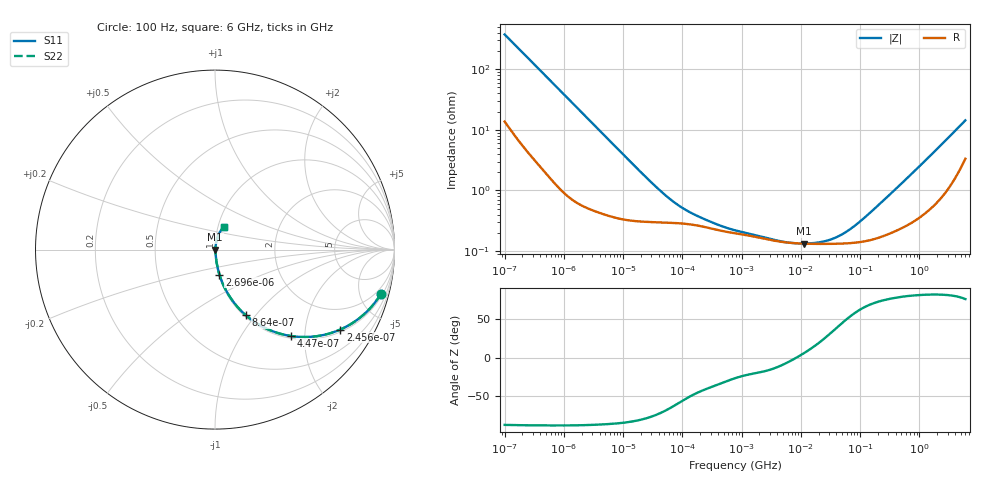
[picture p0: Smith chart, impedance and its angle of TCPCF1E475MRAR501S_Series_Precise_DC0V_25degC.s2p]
! TCPCF1E475MRAR501S Polymer Tantalum Capacitor Sparameter Model
! Model Generated by Samsung Electro-Mechanics
! Samsung Sparameter Version 5.0
! Date : Oct-10-2024
! Products : Polymer Tantalum Capacitor
! Characteristics :
!  Nominal Capacitance = 4.7uF
!  Capacitance Tolerance = +/-20%
!  ESR = 500 mohm max at 100kHz
!  Rated Voltage = 25Vdc
!  Size = 0805(unit:inch), 2012(unit:mm)
!  Length = 2.00+/-0.20mm
!  Width = 1.25+/-0.20mm
!  Thickness = 0.90+/-0.10mm
!  Lineup = Conductive Polymer Type
!  Feature = PCF
!  Measurement Temperature : 25degC.
!  DC bias Value = 0V
!  Frequency : 100Hz ~ 6GHz
! External Node Assignments :
!  1  o---||---o  2
# MHz S RI R 50.0
! Freq.  Real(S11)  Im(S11)  Real(S12)  Im(S12)  Real(S21)  Im(S21)  Real(S22)  Im(S22)
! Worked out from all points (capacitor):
!   300 points, 100 Hz to 6 GHz, reference 50 ohm
!   read as one part in series: C = 4.25 uF near 106.2 Hz
!   lowest |Z| = 134 mohm at 11.14 MHz (marker M1)
!   series resonance near 8.441 MHz, so ESL is about 84 pH
!   S11 on the Smith chart (normalised r, x): 100 Hz: 1.27, -7.44; 245.6 Hz: 1.09, -3.08; 447 Hz: 1.04, -1.71; 864 Hz: 1.02, -0.89; 2.696 kHz: 1.01, -0.29; 6 GHz: 1.07, +0.28
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0.0001  0.9248 -0.2459  0.0752 0.2459  0.0752 0.2459  0.9248 -0.2459
0.0001614771  0.8365 -0.3547  0.1635 0.3547  0.1635 0.3547  0.8365 -0.3547
0.0002455886  0.6982 -0.4454  0.3018 0.4454  0.3018 0.4454  0.6982 -0.4454
0.0004470407  0.4231 -0.4816  0.5769 0.4816  0.5769 0.4816  0.4231 -0.4816
0.0008639723  0.1709 -0.3648  0.8291 0.3648  0.8291 0.3648  0.1709 -0.3648
0.001998454  0.0411 -0.1844  0.9589 0.1844  0.9589 0.1844  0.0411 -0.1844
0.002696271  0.0249 -0.1394  0.9751 0.1394  0.9751 0.1394  0.0249 -0.1394
0.00792526  0.0059 -0.049  0.9941 0.049  0.9941 0.049  0.0059 -0.049
0.03993819  0.00308 -0.00996  0.9969 0.00996  0.9969 0.00996  0.00308 -0.00996
0.0726988  0.00294 -0.00567  0.9971 0.00567  0.9971 0.00567  0.00294 -0.00567
0.1323324  0.00278 -0.00341  0.9972 0.00341  0.9972 0.00341  0.00278 -0.00341
0.366355  0.00227 -0.00166  0.9977 0.00166  0.9977 0.00166  0.00227 -0.00166
0.7981464  0.00196 -0.000977  0.998 0.000977  0.998 0.000977  0.00196 -0.000977
4.534038  0.00143 -0.000269  0.9986 0.000269  0.9986 0.000269  0.00143 -0.000269
11.13508  0.00133 0.000129  0.9987 -0.000129  0.9987 -0.000129  0.00133 0.000129
15.95059  0.00132 0.000316  0.9987 -0.000316  0.9987 -0.000316  0.00132 0.000316
30.82687  0.00132 0.000791  0.9987 -0.000791  0.9987 -0.000791  0.00132 0.000791
56.11362  0.00134 0.00152  0.9987 -0.00152  0.9987 -0.00152  0.00134 0.00152
108.4479  0.00144 0.00296  0.9986 -0.00296  0.9986 -0.00296  0.00144 0.00296
318.7652  0.00202 0.00834  0.998 -0.00834  0.998 -0.00834  0.00202 0.00834
1810.813  0.00759 0.043  0.9924 -0.043  0.9924 -0.043  0.00759 0.043
6000  0.0495 0.128  0.9505 -0.128  0.9505 -0.128  0.0495 0.128
